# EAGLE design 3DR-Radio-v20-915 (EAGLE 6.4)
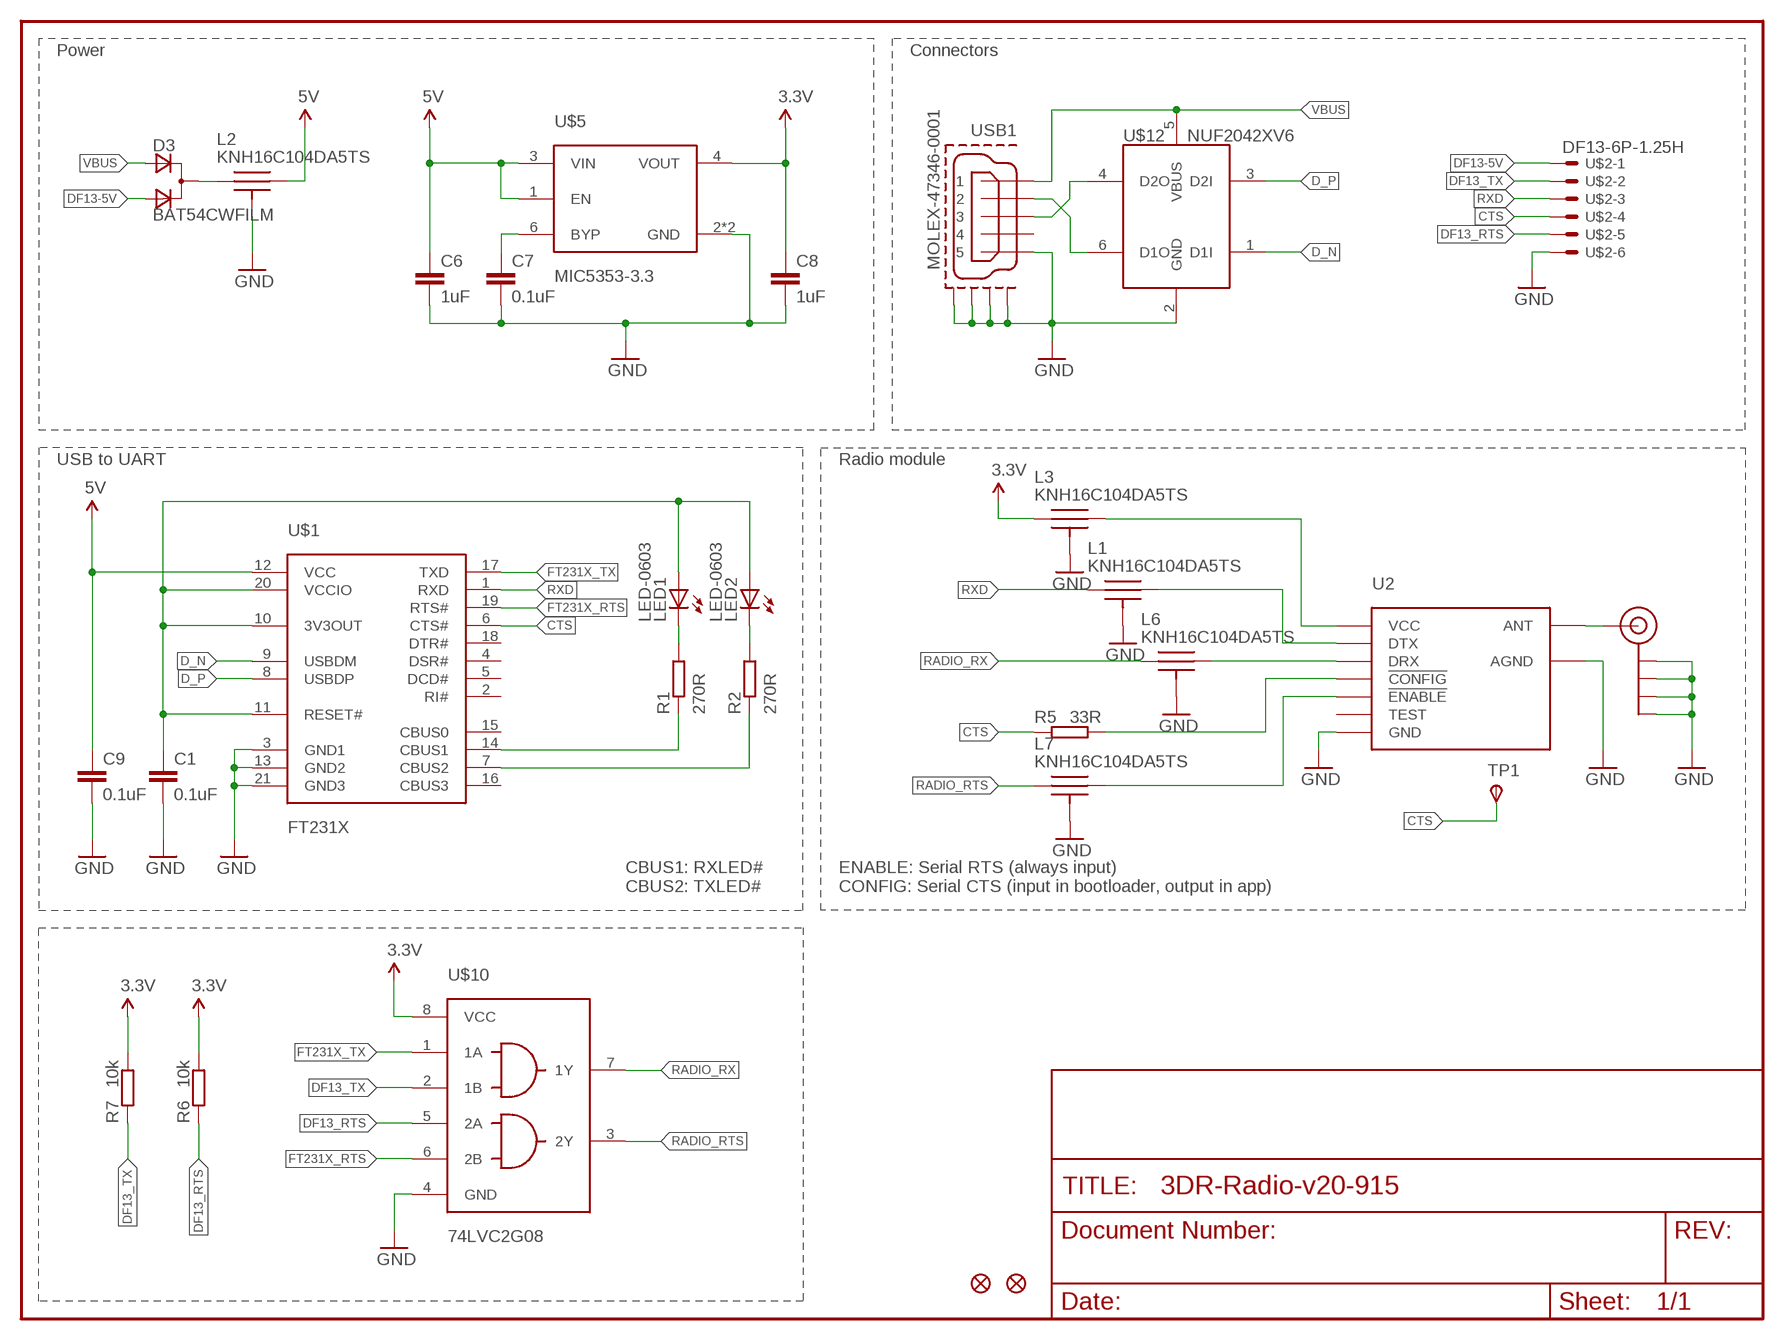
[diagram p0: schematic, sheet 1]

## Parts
C1  0.1uF  CAPACITOR-0402  [0402-CAP]
C6  1uF  CAPACITOR-0402  [0402-CAP]
C7  0.1uF  CAPACITOR-0402  [0402-CAP]
C8  1uF  CAPACITOR-0402  [0402-CAP]
C9  0.1uF  CAPACITOR-0402  [0402-CAP]
D3  BAT54CWFILM  D_2ASOT323  [SOT323]
J$1  SMA_EDGE  [SMA-EDGE]
JP1  FIDUCIAL1X2  [FIDUCIAL-1X2]
JP2  FIDUCIAL1X2  [FIDUCIAL-1X2]
L1  KNH16C104DA5TS  [KYOCERA-KNH16-DA]
L2  KNH16C104DA5TS  [KYOCERA-KNH16-DA]
L3  KNH16C104DA5TS  [KYOCERA-KNH16-DA]
L6  KNH16C104DA5TS  [KYOCERA-KNH16-DA]
L7  KNH16C104DA5TS  [KYOCERA-KNH16-DA]
LED1  LED-0603  [0603-LED]
LED2  LED-0603  [0603-LED]
R1  270R  RESISTOR-0402  [0402-RES]
R2  270R  RESISTOR-0402  [0402-RES]
R5  33R  RESISTOR-0402  [0402-RES]
R6  10k  RESISTOR-0402  [0402-RES]
R7  10k  RESISTOR-0402  [0402-RES]
TP1  TPSTP12R  [TP12R]
U2  HM-TRPSMD  [HM-TRP-SMD]
U$1  FT231X  [QFN20]
U$2  DF13-6P-1.25H  [DF13A-6P-1.25H]
U$5  MIC5353-3.3  MIC5353  [MLF-6-1.6MM]
U$10  74LVC2G08  [VFSOP-8]
U$12  NUF2042XV6  [SOT563-6]
USB1  MOLEX-47346-0001  [MOLEX-47346-0001]

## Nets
3.3V: C8.P$1 L3.P$1 R6.P$1 R7.P$1 U$5.4(VOUT) U$10.8(VCC)
5V: C6.P$1 C9.P$1 L2.P$2 U$1.12(VCC) U$5.1(EN) U$5.3(VIN)
CTS: R5.P$2 TP1.TP(PP) U$1.6(CTS#) U$2.4
D_N: U$1.9(USBDM) U$12.1(D1I)
D_P: U$1.8(USBDP) U$12.3(D2I)
DF13-5V: D3.3(A2) U$2.1
DF13_RTS: R6.P$2 U$2.5 U$10.5(2A)
DF13_TX: R7.P$2 U$2.2 U$10.2(1B)
FT231X_RTS: U$1.19(RTS#) U$10.6(2B)
FT231X_TX: U$1.17(TXD) U$10.1(1A)
GND: C1.P$2 C6.P$2 C7.P$2 C8.P$2 C9.P$2 J$1.GND@0(GND) J$1.GND@1(GND) J$1.GND@2(GND) J$1.GND@3(GND) L1.P$3 L1.P$4 L1.P$5 L2.P$3 L2.P$4 L2.P$5 L3.P$3 L3.P$4 L3.P$5 L6.P$3 L6.P$4 L6.P$5 L7.P$3 L7.P$4 L7.P$5 U2.AGND U2.GND U$1.3(GND1) U$1.13(GND2) U$1.21(GND3) U$2.6 U$5.2(GND) U$5.GNDPAD(GND) U$10.4(GND) U$12.2(GND) USB1.GND USB1.GND1 USB1.GND2 USB1.GND3 USB1.GND4
N$1: J$1.SIG(SIGNAL) U2.ANT
N$2: U$12.6(D1O) USB1.D-
N$3: R1.P$1 U$1.14(CBUS1)
N$4: L1.P$2 U2.DTX
N$5: R2.P$1 U$1.7(CBUS2)
N$6: LED1.C R1.P$2
N$7: L6.P$2 U2.DRX
N$8: LED2.C R2.P$2
N$9: R5.P$1 U2.!CONFIG
N$10: D3.1(C) L2.P$1
N$11: U$12.4(D2O) USB1.D+
N$12: L7.P$2 U2.!ENABLE
N$14: C1.P$1 LED1.A LED2.A U$1.10(3V3OUT) U$1.11(RESET#) U$1.20(VCCIO)
N$16: C7.P$1 U$5.6(BYP)
RADIO_RTS: L7.P$1 U$10.3(2Y)
RADIO_RX: L6.P$1 U$10.7(1Y)
RXD: L1.P$1 U$1.1(RXD) U$2.3
VBUS: D3.2(A1) U$12.5(VBUS) USB1.VBUS
VCC: L3.P$2 U2.VCC
Unconnected: U2.TEST U$1.2(RI#) U$1.4(DSR#) U$1.5(DCD#) U$1.15(CBUS0) U$1.16(CBUS3) U$1.18(DTR#) USB1.ID

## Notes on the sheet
- Power | Connectors
- USB to UART | Radio module
- CBUS1: RXLED#
  CBUS2: TXLED#
- ENABLE: Serial RTS (always input)
  CONFIG: Serial CTS (input in bootloader, output in app)

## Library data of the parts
C1 C6-C9 = pel_dipol_comp:CAPACITOR
D3 = zetex:D_2A: Dual DIODE; OC_FARNELL: unknown; OC_NEWARK: unknown
J$1 = 3DRobotics:SMA_EDGE: SMA Antenna Connector End launch SMA connector. The paste layer has been removed so that the connector can be hand soldered onto the board after reflow.
JP1 JP2 = SparkFun:FIDUCIAL: Fiducial Alignment Points
L1-L3 L6 L7 = pixhawk2:KNH16C104DA5TS: Kyocera KNH16C104DA5TS EMI filter
LED1 LED2 = pel_dipol_comp:LED
R1 R2 R5-R7 = pel_dipol_comp:RESISTOR
TP1 = testpad:TPS: TEST PIN
U2 = 3DRobotics:HM-TRP: HM-TRP Series 100mW Transceiver module HM-TRP series is a low cost, high performance transparent FSK transceiver with operating at 433/470/868/915 MHz. It features small size, high output power, high sensitivity, long transmission distance and high communication data rate with auto set up for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
U$1 = 3DRobotics:FT231X: FT231X – Full Speed USB to Full Handshake UART This USB2.0 Full Speed IC offers a compact bridge to full handshake UART interfaces. The device is a UART, capable of operating up to 3MBaud, with low power consumption (8mA). The FT231X includes the complete FT-X series feature set and enables USB to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; DATASHEET: http://www.ftdichip.com/Support/Documents/DataSheets/ICs/DS_FT231X.pdf; LINK: http://www.ftdichip.com/Products/ICs/FT231X.html; MFGPN: FT231X
U$2 = pixhawk2:DF13-6P-1.25?
U$5 = 3DRobotics:MIC5353: MIC5353 - 500mA LDO in 1.6mm × 1.6mm Package The MIC5353 is a high-performance, single-output, ultra- low LDO (ULDOTM) regulator, offering a low total output noise of 30μVRMS. The MIC5353 is capable of sourcing 500mA output current and offers high-PSRR and low- output noise, making it an ideal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; DATASHEET: http://www.micrel.com/_PDF/mic5353.pdf; LINK: http://www.micrel.com/index.php/en/products/power-management-ics/ldos/single-ldos/article/79-mic5353-.html; MFGPN: MIC5353
U$10 = 3DRobotics:74LVC2G08: 74LVC2G08 dual 2-input AND gate Inputs can be driven from either 3.3 V or 5 V devices. This feature allows the use of the 74LVC2G08 as a translator in a mixed 3.3 V and 5 V environment. This device is fully specified for partial power-down applications using IOFF. The IOFF circuitry disables the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; DATASHEET: http://www.nxp.com/documents/data_sheet/74LVC2G08.pdf; LINK: http://www.nxp.com/products/logic/gates/and_gates/74LVC2G08DC.html; MFGPN: 74LVC2G08
U$12 = pixhawk2:NUF2042XV6
USB1 = pixhawk2:MOLEX-47346-0001: MICRO USB B, BOTTOM MOUNT

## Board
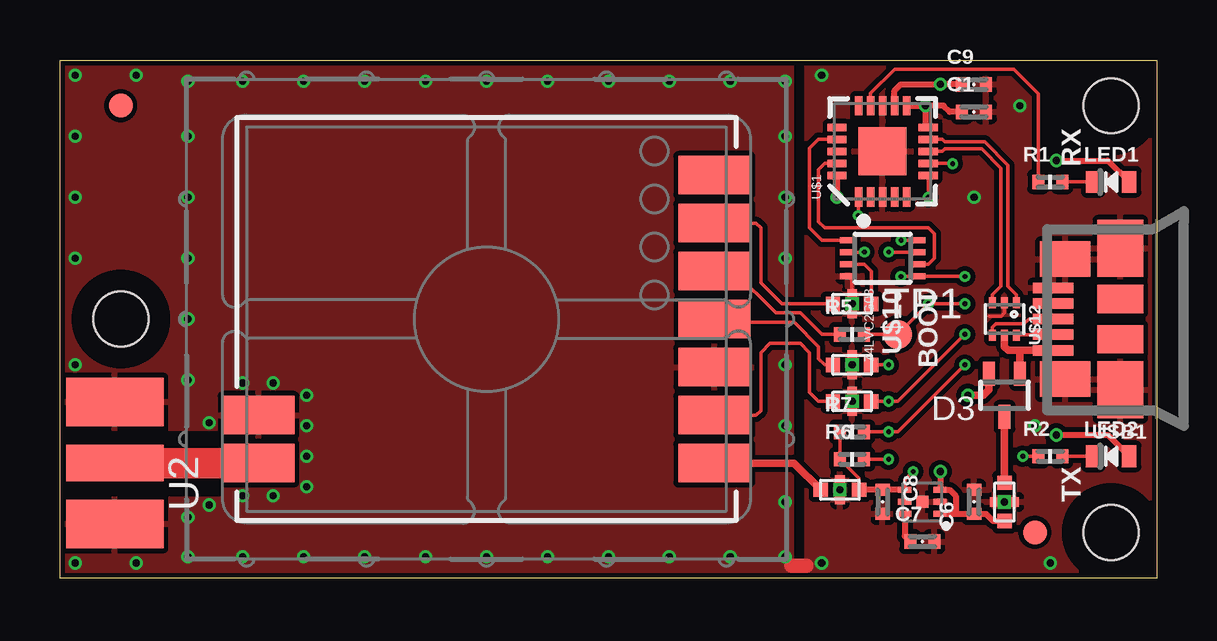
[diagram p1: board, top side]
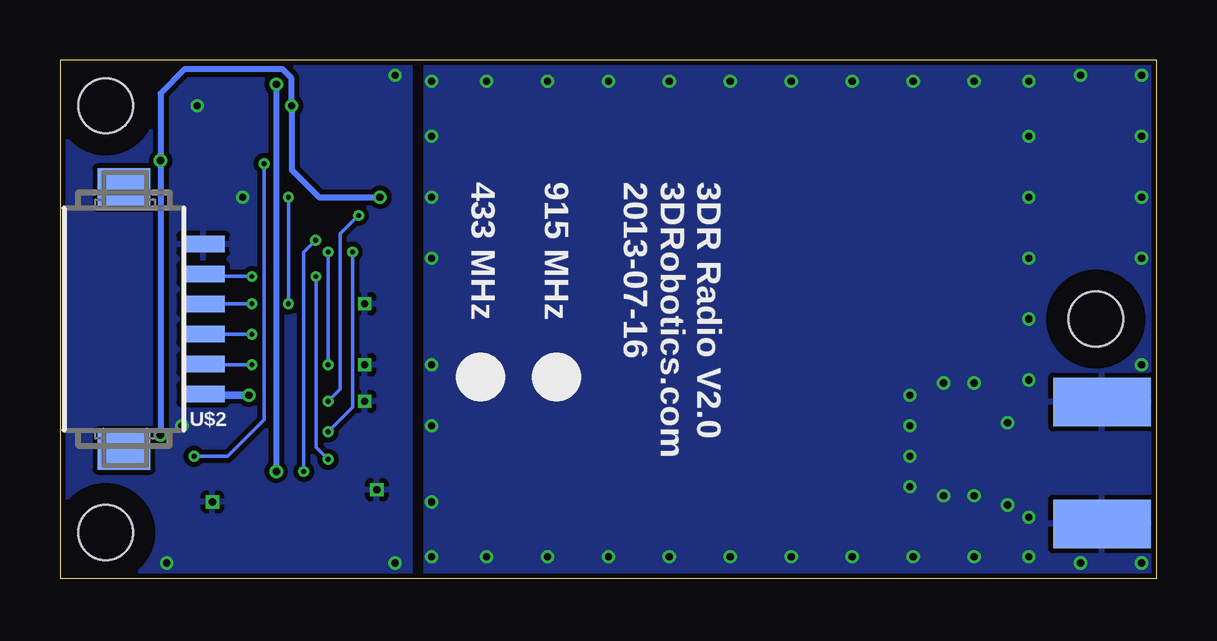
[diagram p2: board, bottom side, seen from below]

Size 45.72 x 21.59 mm. Coordinates in mm from the lower left corner, seen from the top.
Outline: 0,0 0,21.59 45.72,21.59 45.72,0 0,0
Copper layers (1*2*3*14*15*16): Top 0.035mm / dielectric 0.5mm / Route2 0.035mm / dielectric 0.15mm / Route3 0.035mm / dielectric 0.15mm / Route14 0.035mm / dielectric 0.15mm / Route15 0.035mm / dielectric 0.5mm / Bottom 0.035mm
Design rules "PX4FMUv2": minimum track width 0.15mm, minimum drill 0.2mm, track to track 0.15mm, track to pad 0.15mm, pad to pad 0.15mm, via to via 0.15mm, smd to smd 0.15mm, copper to edge 0.2mm, drill to drill 0.2mm, minimum pad ring 0.125mm, minimum via ring 0.125mm, stop-mask expansion 1mil, vias tented up to drill 0.31mm, thermal gap 8mil
Holes 2.29 mm at 2.54,10.79 43.81,19.68 43.81,1.91
tKeepout: area 0.8,9 to 4.3,12.6; area 42,17.9 to 45.6,21.5; area 42,0.1 to 45.6,3.7
tRestrict: area 0.8,9 to 4.3,12.6; area 42,17.9 to 45.6,21.5; area 42,0.1 to 45.6,3.7
bRestrict: area 0.8,9 to 4.3,12.6; area 42,17.9 to 45.6,21.5; area 42,0.1 to 45.6,3.7

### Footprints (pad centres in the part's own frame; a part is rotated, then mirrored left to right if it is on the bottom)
0402-CAP = smd 0.5 x 0.6: P$1 -0.5,0; P$2 0.5,0
SOT323 = smd 0.5 x 1: 1 0,0.9; 2 -0.65,-0.9; 3 0.65,-0.9
SMA-EDGE = smd 2.032 x 4.064: GND@0 -2.54,0; GND@1 2.54,0 | smd 2.032 x 4.064 bottom: GND@2 -2.54,0; GND@3 2.54,0 | smd 1.524 x 4.064: SIG 0,0
FIDUCIAL-1X2 = smd 1 x 1: 1 0,0
KYOCERA-KNH16-DA = smd 0.6 x 0.6: P$1 -0.8,0; P$2 0.8,0 | smd 0.4 x 0.4: P$3 0,-0.4; P$4 0,0.4 | drill 0.3 pad 0.4 square: P$5 0,0
0603-LED = smd 0.6 x 0.9: A 0.75,0; C -0.75,0
0402-RES = smd 0.5 x 0.6: P$1 -0.5,0; P$2 0.5,0
TP12R = smd 1.2 x 1.2: TP 0,0
HM-TRP-SMD = smd 1.6 x 3: !CONFIG 2,-9.5; !ENABLE 4,-9.5; AGND -4,9.5; ANT -6,9.5; DRX 0,-9.5; DTX -4,-9.5; GND -2,-9.5; TEST 6,-9.5; VCC -6,-9.5
QFN20 = smd 0.8 x 0.3: 1 -1.9,1; 2 -1.9,0.5; 3 -1.9,0; 4 -1.9,-0.5; 5 -1.9,-1; 11 1.9,-1; 12 1.9,-0.5; 13 1.9,0; 14 1.9,0.5; 15 1.9,1 | smd 0.3 x 0.8: 6 -1,-1.9; 7 -0.5,-1.9; 8 0,-1.9; 9 0.5,-1.9; 10 1,-1.9; 16 1,1.9; 17 0.5,1.9; 18 0,1.9; 19 -0.5,1.9; 20 -1,1.9 | smd 2 x 2: 21 0,0
DF13A-6P-1.25H = smd 0.7 x 1.8: 1 -3.125,-3.3; 2 -1.875,-3.3; 3 -0.625,-3.3; 4 0.625,-3.3; 5 1.875,-3.3; 6 3.125,-3.3 | smd 1.6 x 2.2: S1 5.475,0; S2 -5.475,0
MLF-6-1.6MM = smd 0.25 x 0.55: 1 -0.5,-0.73; 2 0,-0.73; 3 0.5,-0.73; 4 0.5,0.73; 5 0,0.73; 6 -0.5,0.73 | smd 0.5 x 0.5: GNDPAD 0,0
VFSOP-8 = smd 0.25 x 0.65: 1 -0.75,-1.45; 2 -0.25,-1.45; 3 0.25,-1.45; 4 0.75,-1.45; 5 0.75,1.45; 6 0.25,1.45; 7 -0.25,1.45; 8 -0.75,1.45
SOT563-6 = smd 0.3 x 0.45: 1 -0.5,-0.675; 2 0,-0.675; 3 0.5,-0.675; 4 0.5,0.675; 5 0,0.675; 6 -0.5,0.675
MOLEX-47346-0001 = smd 1.7 x 0.44: D+ 2.8,0; D- 2.8,0.65; GND 2.8,-1.3; ID 2.8,-0.65; VBUS 2.8,1.3 | smd 1.9 x 2.375: GND1 0,2.95; GND4 0,-2.95 | smd 2.1 x 1.475: GND2 2.3,2.5; GND3 2.3,-2.5 | smd 1.9 x 1.175: GND5 0,-0.838; GND6 0,0.838

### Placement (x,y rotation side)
C1  38.1,19.43 0 top
C6  38.1,3.17 90 top
C7  35.94,1.52 0 top
C8  34.29,3.17 270 top
C9  38.1,20.57 0 top
D3  39.37,7.62 180 top
J$1  2.29,4.8 90 top
JP1  40.64,1.91 0 top
JP2  2.54,19.68 0 top
L1  33.02,7.37 180 top
L2  39.37,3.17 270 top
L3  32.51,3.68 180 top
L6  33.02,8.89 180 top
L7  33.02,11.43 180 top
LED1  43.81,16.51 0 top
LED2  43.81,5.08 0 top
R1  41.27,16.51 0 top
R2  41.27,5.08 0 top
R5  33.02,10.16 0 top
R6  33.02,4.95 0 top
R7  33.02,6.1 0 top
TP1  34.92,10.16 0 top
U2  17.78,10.79 90 top
U$1  34.29,17.78 90 top
U$2  43.05,10.79 90 bottom
U$4  [3DR-EMI-SHIELD-25X20]  17.78,10.79 0 top
U$5  35.94,3.17 90 top
U$10  34.29,13.34 270 top
U$12  39.37,10.79 180 top
USB1  44.2,10.79 180 top

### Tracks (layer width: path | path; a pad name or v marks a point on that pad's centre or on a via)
3.3V  (via drill 0.2)
  Top 0.152: R7.P$1 R6.P$1 33.31,4.16 L3.P$1 | U$10.8 v35.06,14.09 v35.05,14.1 | U$5.4 35.21,4.1 v35.56,4.45
  Top 0.254: U$5.4 C8.P$1 L3.P$1
  Bottom 0.152: v35.06,14.09 35.56,13.59 v35.56,4.45
5V  (via drill 0.3)
  Top 0.254: U$1.12 34.79,20.31 35.05,20.57 v36.7,20.57 C9.P$1 | U$5.1 37.34,2.67 | 37.34,2.67 C6.P$1 38.6,2.67 38.9,2.38 L2.P$2 | 37.34,2.67 37.34,3.43 37.09,3.67 U$5.3 36.7,3.71 v36.7,4.45
  Bottom 0.254: v36.7,20.57 v36.7,4.45
CTS  (via drill 0.2)
  Top 0.152: U$1.6 v36.19,15.88 v36.2,15.88 | v37.72,11.43 v36.2,11.43 TP1.TP R5.P$2
  Bottom 0.152: v36.2,15.88 v36.2,11.43 | v37.72,11.43 U$2.4
D_N
  Top 0.15: U$1.9 36.78,18.28 36.88,18.18 38.54,18.18 39.52,17.21 39.52,12.17 39.87,11.82 U$12.1
D_P
  Top 0.15: U$1.8 36.78,17.78 36.88,17.88 38.42,17.88 39.22,17.08 39.22,12.17 38.87,11.82 U$12.3
DF13-5V  (via drill 0.3)
  Top 0.305: v37.85,7.62 38.48,7.62 38.72,7.86 D3.3
  Bottom 0.305: v37.85,7.62 39.7,7.62 U$2.1
DF13_RTS  (via drill 0.2)
  Top 0.152: v37.72,12.57 37.71,12.59 U$10.5 35.06,12.59 v35.05,12.57 | R6.P$2 v34.54,4.95
  Bottom 0.152: v37.72,12.57 39.66,12.57 U$2.5 | v35.05,12.57 35.05,5.46 v34.54,4.95
DF13_TX  (via drill 0.2)
  Top 0.152: v33.53,13.59 U$10.2 | R7.P$2 v34.54,6.1 34.92,6.1 v37.72,8.89
  Bottom 0.152: v37.72,8.89 39.72,8.89 U$2.2 | v33.53,13.59 33.53,7.11 v34.54,6.1
FT231X_RTS
  Top 0.152: U$1.19 31.89,17.28 31.62,17.02 31.62,14.86 31.88,14.61 36.2,14.61 36.45,14.35 36.45,13.34 36.2,13.09 U$10.6
FT231X_TX
  Top 0.152: U$1.17 31.61,18.28 31.24,17.91 31.24,14.61 31.76,14.09 U$10.1
GND  (via drill 0.3)
  Top 0.152: L7.P$3 33.02,12.4 U$10.4 | U$12.2 39.37,11.05 39.24,10.92 38.73,10.92
  Top 0.61: 30.48,0.51 31.11,0.51
  other vias: 5.33,20.7 5.33,18.41 5.33,15.88 5.33,13.34 5.33,10.79 5.33,2.54 5.33,0.89 15.24,0.89 7.62,20.7 10.16,20.7 12.7,20.7 15.24,20.7 17.78,20.7 20.32,20.7 30.23,20.7 30.23,18.41 30.23,15.88 30.23,3.17 30.23,0.89 27.94,0.89 25.4,0.89 22.86,0.89 20.32,0.89 17.78,0.89 5.33,8.26 22.86,20.7 25.4,20.7 27.94,20.7 12.7,0.89 10.16,0.89 7.62,0.89 0.64,8.89 0.64,13.34 0.64,15.88 0.64,18.41 0.64,20.95 3.17,20.95 0.64,0.64 3.17,0.64 30.23,13.34 30.23,8.89 30.23,6.35 6.22,3.05 6.22,6.48 7.62,3.43 8.89,3.43 10.29,3.81 10.29,5.08 10.29,6.35 10.29,7.62 8.89,8.13 7.62,8.13 40.01,19.68 41.27,0.64 31.75,0.64 31.75,20.95 38.1,15.88 40.64,6.35
  pour Top (isolate 0.203): -0.64,-0.64 -0.64,3.3 6.86,3.3 6.86,6.22 -0.64,6.22 -0.64,22.23 30.48,22.23 30.48,-0.64
  pour Bottom (isolate 0.203): -1.27,-1.27 -1.27,22.86 30.48,22.86 30.48,-1.27
  pour Top (isolate 0.203): 31.11,22.23 31.11,-0.64 46.35,-0.64 46.35,22.23
  pour Bottom (isolate 0.203): 31.11,-1.27 31.11,22.86 46.99,22.86 46.99,-1.27
N$1
  Top 1.27: U2.ANT 2.19,4.79 J$1.SIG
N$2
  Top 0.152: USB1.D- 39.9,10.14 U$12.6
N$3
  Top 0.152: U$1.14 33.79,20.2 34.8,21.21 39.75,21.21 40.77,20.18 R1.P$1
N$4
  Top 0.152: U2.DTX 29.02,6.79 29.21,6.99 29.21,9.4 29.59,9.78 30.86,9.78 31.24,9.4 31.24,7.75 31.62,7.37 L1.P$2
N$5  (via drill 0.2)
  Top 0.152: v40.13,5.08 R2.P$1 | U$1.7 v37.2,17.28 v37.21,17.27
  Bottom 0.152: v37.21,17.27 37.21,6.6 38.73,5.08 v40.13,5.08
N$6
  Top 0.152: LED1.C R1.P$2
N$7
  Top 0.152: U2.DRX 27.41,10.67 30.61,10.67 31.62,9.65 31.62,9.14 31.88,8.89 L6.P$2
N$8
  Top 0.152: LED2.C R2.P$2
N$9
  Top 0.152: U2.!CONFIG 28.1,12.79 29.84,11.05 30.86,11.05 31.75,10.16 R5.P$1
N$10
  Top 0.305: D3.1 L2.P$1
N$11
  Top 0.152: USB1.D+ 40.39,10.79 40.18,10.59 39.01,10.59 38.87,10.45 U$12.4
N$12
  Top 0.152: U2.!ENABLE 29.02,14.79 29.21,14.61 29.21,12.32 30.1,11.43 L7.P$2
N$14  (via drill 0.3)
  Top 0.254: C1.P$1 37.08,19.43 36.83,19.68 v36.07,19.68 | U$1.20 v32.39,15.88 v32.38,15.88 | U$1.11 v36.07,19.68 | v36.07,19.68 36.07,18.9 U$1.10 | v41.53,17.4 43.68,17.4 LED1.A | v41.53,5.97 43.68,5.97 LED2.A
  Bottom 0.254: v32.38,15.88 34.92,15.88 36.06,17.01 v36.06,19.68 v36.07,19.68 36.07,20.83 36.45,21.21 40.51,21.21 41.53,20.19 v41.53,17.4 v41.53,5.97
N$16
  Top 0.254: U$5.6 35.21,1.75 C7.P$1
RADIO_RTS
  Top 0.152: L7.P$1 33.82,12.79 33.52,13.09 U$10.3
RADIO_RX  (via drill 0.2)
  Top 0.152: L6.P$1 v34.54,8.89 | U$10.7 v34.55,13.59 v34.54,13.59
  Bottom 0.152: v34.54,13.59 v34.54,8.89
RXD  (via drill 0.2)
  Top 0.152: U$1.1 33.29,15.13 v33.27,15.11 | L1.P$1 v34.54,7.37 34.92,7.37 v37.72,10.16
  Bottom 0.152: v37.72,10.16 U$2.3 | v33.27,15.11 34.04,14.35 34.04,7.87 v34.54,7.37
VBUS
  Top 0.305: USB1.VBUS 40.01,9.49 | 40.01,9.49 39.53,9.49 39.37,9.65 U$12.5 | D3.2 40.02,9.48 40.01,9.49
VCC
  Top 0.305: U2.VCC 30.6,4.79 L3.P$2

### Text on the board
tPlace: RX | BOOT | TX
bPlace: 3DR Radio V2.0 / 3DRobotics.com / 2013-07-16 | 915 MHz / / 433 MHz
